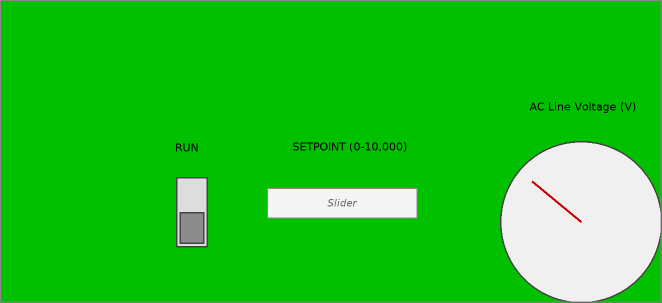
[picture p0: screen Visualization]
VISUALIZATION Visualization  // 662x303
    DipSwitch (157,177 70x70), variable: MAIN.TOGGLE_RUN_ENABLE, behaviour: TOGGLE, style: Switch-DipSwitch-Gray
    Label (112,133 150x30), "RUN"
    Slider (267,188 150x30), variable: MAIN.SETPOINT_PERCENT, scale 0..100
    Label (275,132 150x30), "SETPOINT (0-10,000)"
    Meter360 (500,141 162x162), value: MAIN.AC_LINE_VOLTAGE, style: Meter-Meter360-Gray, scale format: %.1f, scale 0..100
    Label (508,92 150x30), "AC Line Voltage (V)"
END_VISUALIZATION
